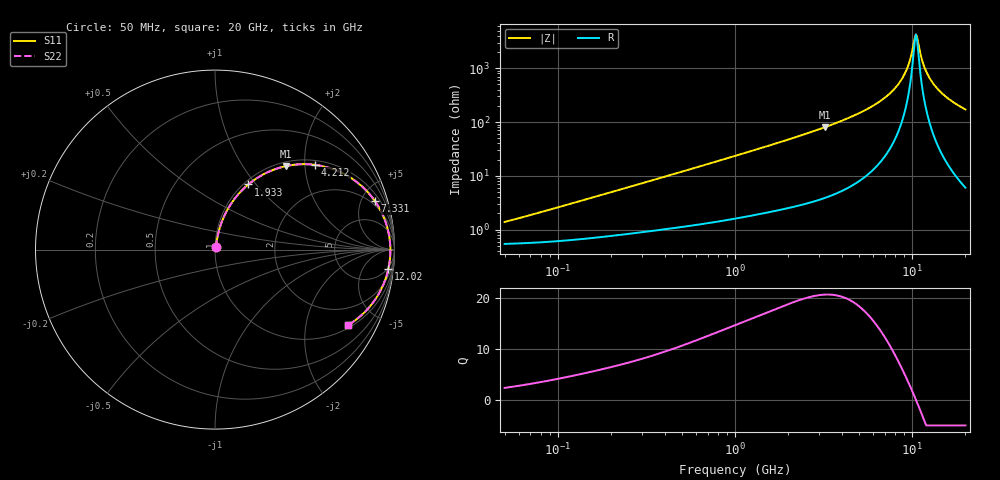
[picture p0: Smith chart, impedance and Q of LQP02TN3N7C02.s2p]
!Murata Part Number: LQP02TN3N7C02
!These Parameters are Measured in Series Mode Connection
!  o--[Z]--o
!Port1  Port2
!  o-------o
!Freq. Start=50[MHz] Stop=20[GHz], 401[Steps]
# Hz S RI R 50
!Freq.(Hz) S11(Real) S11(Imag) S21(Real) S21(Imag) S12(Real) S12(Imag) S22(Real) S22(Imag)
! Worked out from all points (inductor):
!   401 points, 50 MHz to 20 GHz, reference 50 ohm
!   read as one part in series: L = 4.04 nH near 66.46 MHz
!   highest Q = 20.6 at 3.217 GHz (marker M1), where L = 3.97 nH
!   self-resonance near 10.5 GHz
!   S11 on the Smith chart (normalised r, x): 50 MHz: 1.01, +0.03; 1.933 GHz: 1.05, +0.91; 4.212 GHz: 1.11, +2.26; 7.331 GHz: 1.57, +6.37; 12.02 GHz: 4, -17; 20 GHz: 1.12, -3.43
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5e7  0.00557 0.0127  0.9944 -0.0127  0.9944 -0.0127  0.00557 0.0127
1.364002e8  0.00778 0.0336  0.9922 -0.0336  0.9922 -0.0336  0.00778 0.0336
3.721004e8  0.0174 0.0869  0.9826 -0.0869  0.9826 -0.0869  0.0174 0.0869
1e9  0.0654 0.2154  0.9346 -0.2154  0.9346 -0.2154  0.0654 0.2154
1.932977e9  0.1855 0.3627  0.8145 -0.3627  0.8145 -0.3627  0.1855 0.3627
2.728004e9  0.3141 0.4401  0.6859 -0.4401  0.6859 -0.4401  0.3141 0.4401
3.216634e9  0.3968 0.4656  0.6032 -0.4656  0.6032 -0.4656  0.3968 0.4656
4.212059e9  0.5585 0.4721  0.4415 -0.4721  0.4415 -0.4721  0.5585 0.4721
5.769027e9  0.7615 0.3966  0.2385 -0.3966  0.2385 -0.3966  0.7615 0.3966
7.331367e9  0.891 0.2702  0.109 -0.2702  0.109 -0.2702  0.891 0.2702
7.442007e9  0.8975 0.2605  0.1025 -0.2605  0.1025 -0.2605  0.8975 0.2605
8.264682e9  0.9369 0.188  0.0631 -0.188  0.0631 -0.188  0.9369 0.188
9.041845e9  0.9606 0.1204  0.0394 -0.1204  0.0394 -0.1204  0.9606 0.1204
9.600142e9  0.9707 0.0734  0.0293 -0.0734  0.0293 -0.0734  0.9707 0.0734
1.019291e10  0.9761 0.0255  0.0239 -0.0255  0.0239 -0.0255  0.9761 0.0255
1.050288e10  0.977 0.00134  0.023 -0.00134  0.023 -0.00134  0.977 0.00134
1.082228e10  0.9767 -0.0228  0.0233 0.0228  0.0233 0.0228  0.9767 -0.0228
1.149051e10  0.9725 -0.071  0.0275 0.071  0.0275 0.071  0.9725 -0.071
1.201863e10  0.9662 -0.1067  0.0338 0.1067  0.0338 0.1067  0.9662 -0.1067
1.314879e10  0.9458 -0.176  0.0542 0.176  0.0542 0.176  0.9458 -0.176
1.460232e10  0.9095 -0.2513  0.0905 0.2513  0.0905 0.2513  0.9095 -0.2513
2e10  0.7397 -0.4216  0.2603 0.4216  0.2603 0.4216  0.7397 -0.4216
